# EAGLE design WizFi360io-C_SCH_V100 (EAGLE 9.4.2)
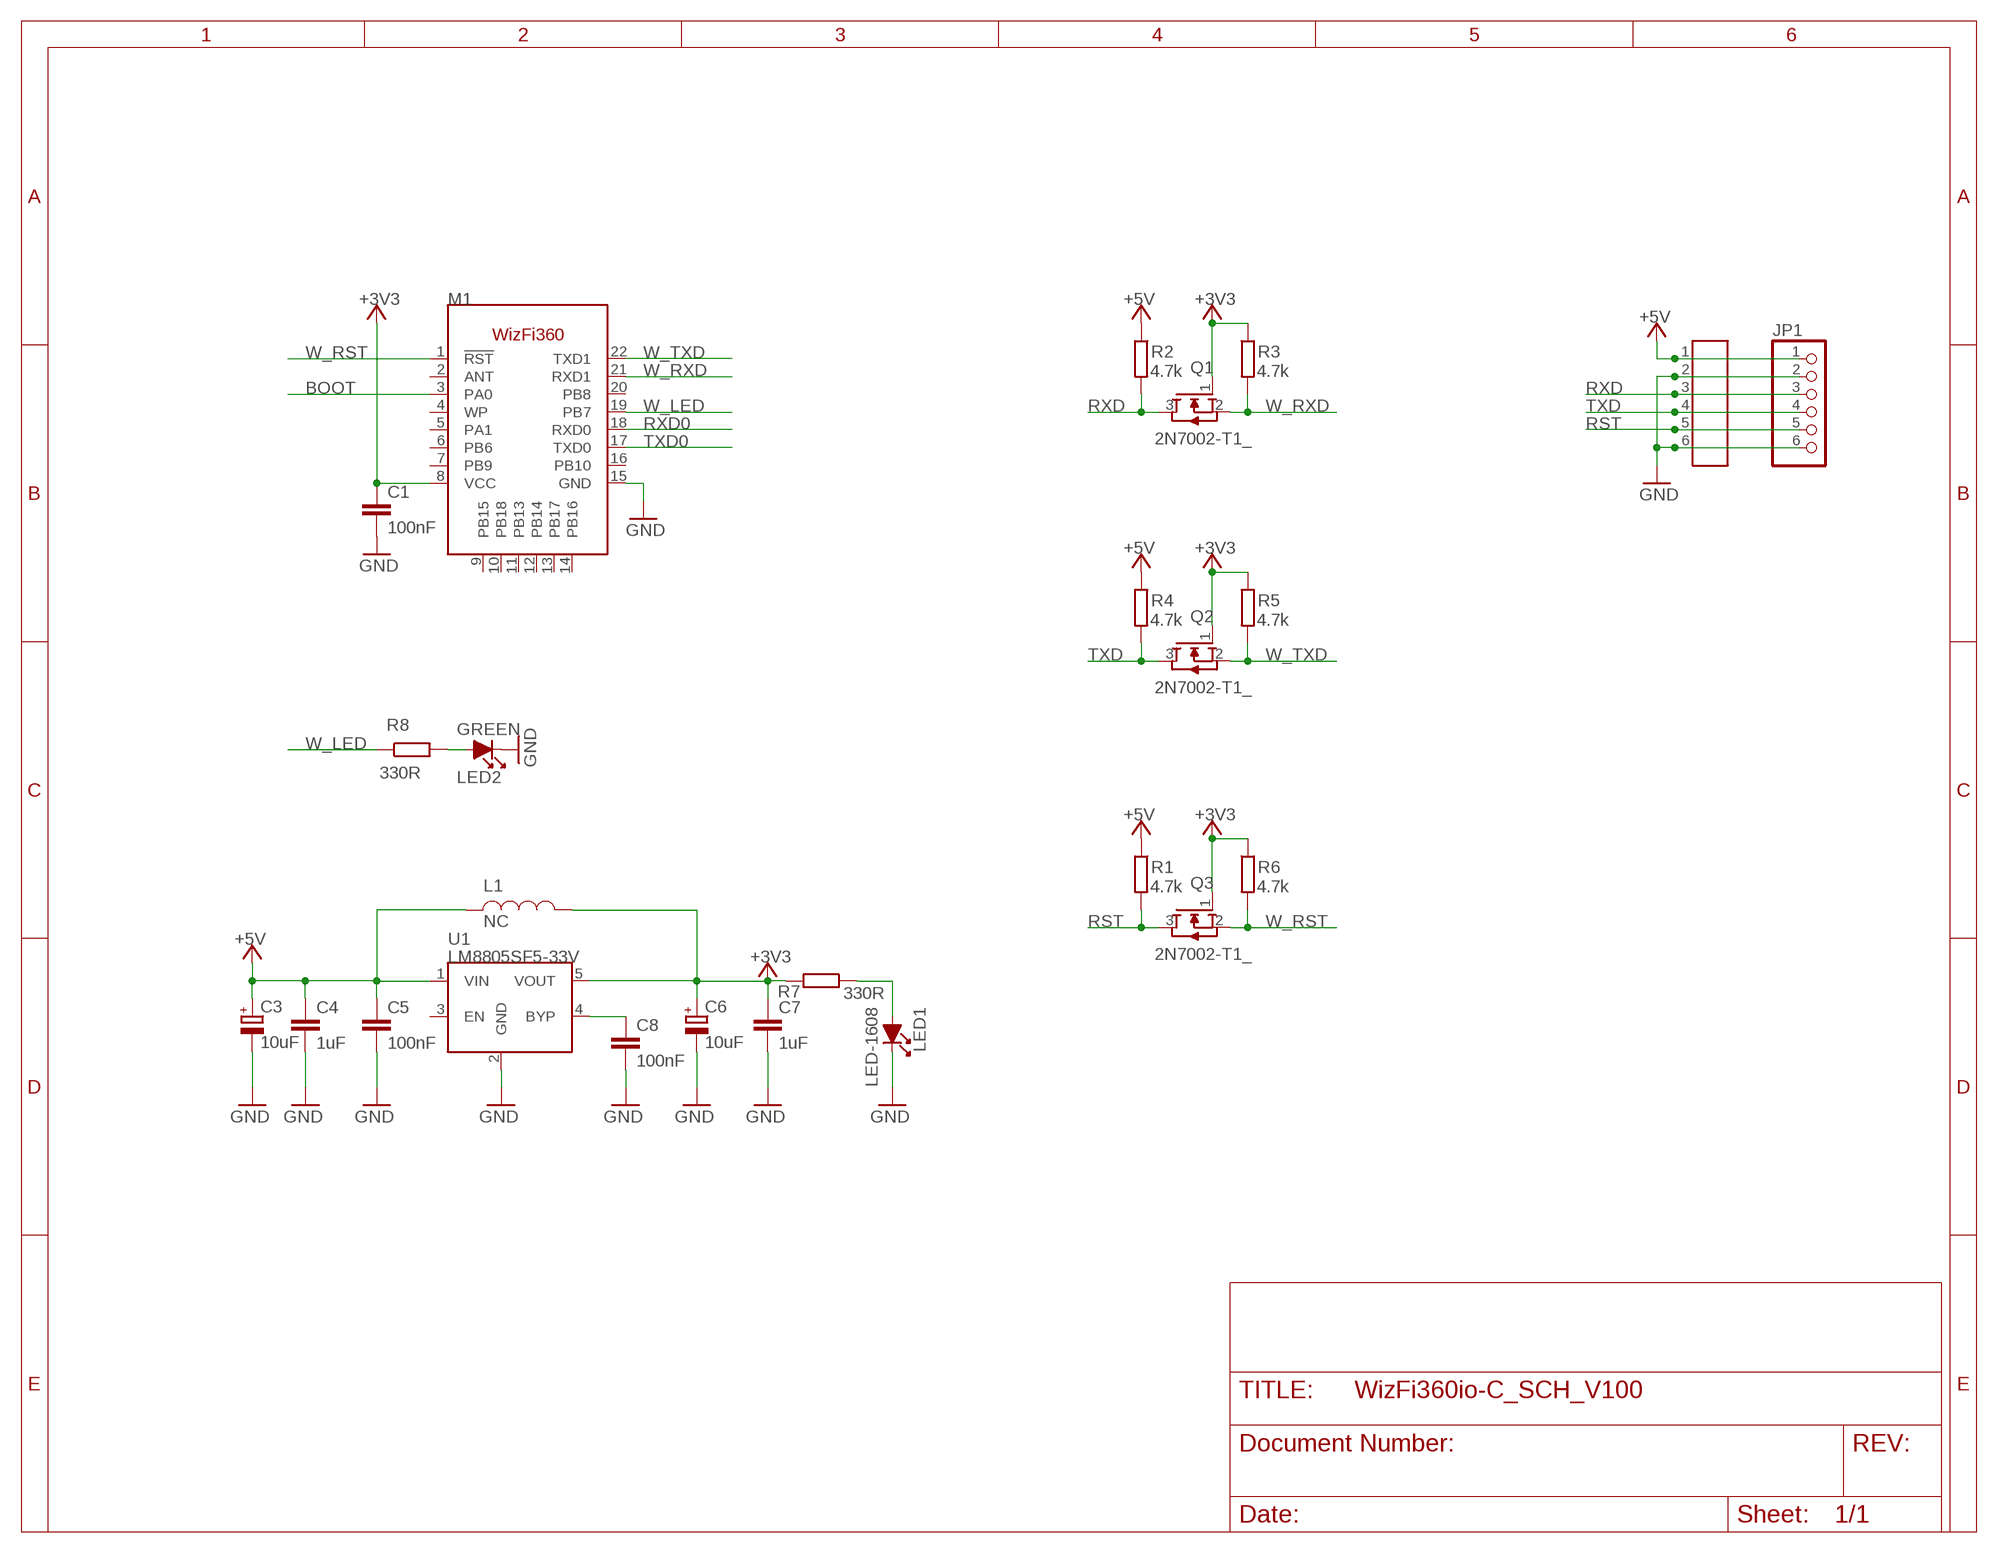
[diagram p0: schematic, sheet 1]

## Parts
C1  100nF  0142_10NF_0603  [C0603-ROUND@1]
C3  10uF  0474_TAJA475M016RNJ  [SMC_A]
C4  1uF  0142_10NF_0603  [C0603-ROUND@1]
C5  100nF  0142_10NF_0603  [C0603-ROUND@1]
C6  10uF  0474_TAJA475M016RNJ  [SMC_A]
C7  1uF  0142_10NF_0603  [C0603-ROUND@1]
C8  100nF  0142_10NF_0603  [C0603-ROUND@1]
JP1  PINHD-1X6NO_SILK  [1X06_NO_SILK]
JP4  SMW200-06  [SMW200-06]
L1  NC  L-1608  [L-1608]
LED1  LED-1608  [LED-1608]
LED2  GREEN  LED-1608  [LED-1608]
M1  WIZFI360  [WIZFI360]
Q1  2N7002-T1_  [SOT23]
Q2  2N7002-T1_  [SOT23]
Q3  2N7002-T1_  [SOT23]
R1  4.7k  0028_CR0603JW103L  [R0603-ROUND]
R2  4.7k  0028_CR0603JW103L  [R0603-ROUND]
R3  4.7k  0028_CR0603JW103L  [R0603-ROUND]
R4  4.7k  0028_CR0603JW103L  [R0603-ROUND]
R5  4.7k  0028_CR0603JW103L  [R0603-ROUND]
R6  4.7k  0028_CR0603JW103L  [R0603-ROUND]
R7  330R  0028_CR0603JW103L  [R0603-ROUND]
R8  330R  0028_CR0603JW103L  [R0603-ROUND]
U1  LM8805SF5-33V  [SOT23-5L]

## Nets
+3V3 [power]: C1.1 C6.+ C7.1 L1.P$2 M1.8(VCC) Q1.1(G) Q2.1(G) Q3.1(G) R3.1 R5.1 R6.1 R7.2 U1.5(VOUT)
+5V: C3.+ C4.1 C5.1 JP1.1 JP4.1 L1.1 R1.1 R2.1 R4.1 U1.1(VIN)
BOOT: M1.3(PA0)
GND: C1.2 C3.- C4.2 C5.2 C6.- C7.2 C8.2 JP1.2 JP1.6 JP4.2 JP4.6 LED1.K LED2.K M1.15(GND) U1.2(GND)
N$2: C8.1 U1.4(BYP)
N$7: LED1.A R7.1
N$17: LED2.A R8.2
RST: JP1.5 JP4.5 Q3.3(D) R1.2
RXD: JP1.3 JP4.3 Q1.3(D) R2.2
RXD0: M1.18(RXD0)
TXD: JP1.4 JP4.4 Q2.3(D) R4.2
TXD0: M1.17(TXD0)
W_LED: M1.19(PB7) R8.1
W_RST: M1.1(!RST!) Q3.2(S) R6.2
W_RXD: M1.21(RXD1) Q1.2(S) R3.2
W_TXD: M1.22(TXD1) Q2.2(S) R5.2
Unconnected: M1.2(ANT) M1.4(WP) M1.5(PA1) M1.6(PB6) M1.7(PB9) M1.9(PB15) M1.10(PB18) M1.11(PB13) M1.12(PB14) M1.13(PB17) M1.14(PB16) M1.16(PB10) M1.20(PB8) U1.3(EN)

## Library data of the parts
C1 C4 C5 C7 C8 = Condensatori:0142_10NF_0603: 10nF 0603; CASE: 0603; MONTHLY_USAGE: _____; PART_NUMBER: 10nF_0603; PRICE: _____; SUPPLIER: _____; TYPE: Condensatori; VALUE: 10nF
C3 C6 = Condensatori:0474_TAJA475M016RNJ: 4u7 tantalio Case A - testa gialla -Tantalio; CASE: CaseA_(1206); MONTHLY_USAGE: _____; PART_NUMBER: TAJA475M016RNJ; PRICE: _____; SUPPLIER: _____; TYPE: Condensatori; VALUE: 4u7
JP1 = PinHeader:PINHD-1X6: PIN HEADER
JP4 = Connector:SMW200-06
L1 = INDUCTOR:L-1608
LED1 LED2 = DIODE:LED-1608
M1 = WIZnet:WIZFI360
Q1-Q3 = TRANSISTOR:2N7002-T1
R1-R8 = Resistenze:0028_CR0603JW103L: 10K 0603; CASE: 0603; MONTHLY_USAGE: _____; PART_NUMBER: CR0603JW103L; PRICE: _____; SUPPLIER: _____; TYPE: Resistenze; VALUE: 10k
U1 = RECULATOR:LM8805SF5-33V

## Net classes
0 default: width 0.203 mm, drill 0.008 mm, clearance 0.127 mm
1 power: width 0.305 mm, drill 0.3 mm, clearance 0.203 mm

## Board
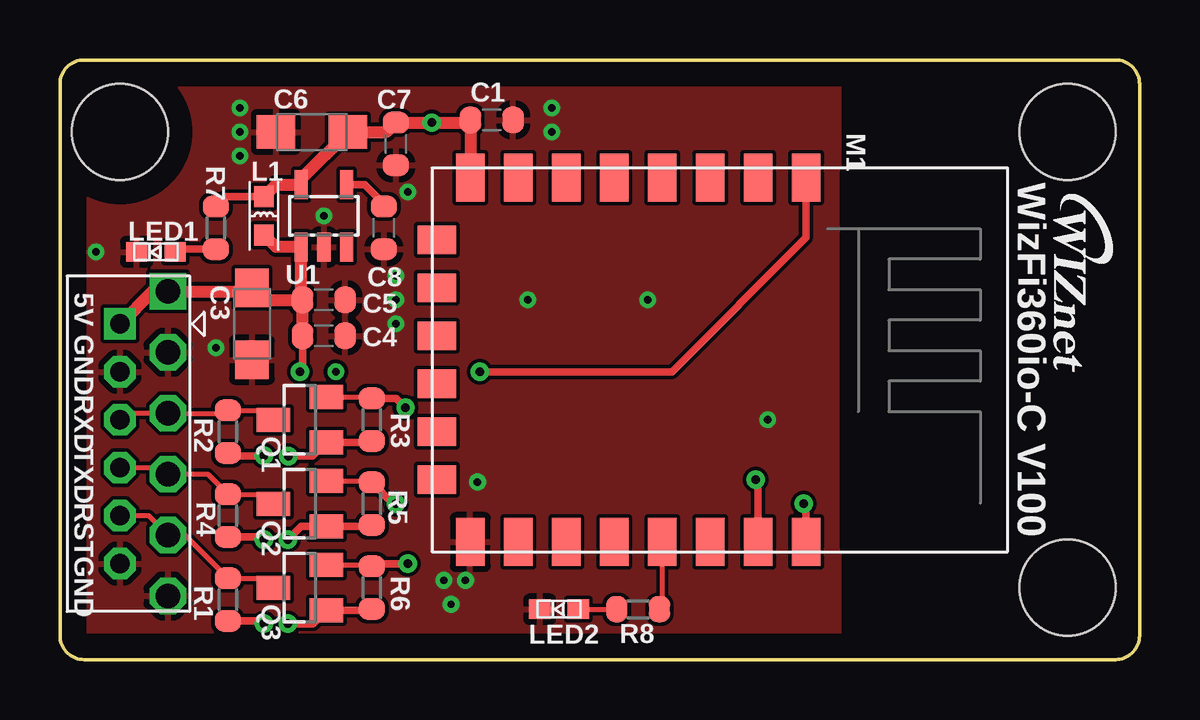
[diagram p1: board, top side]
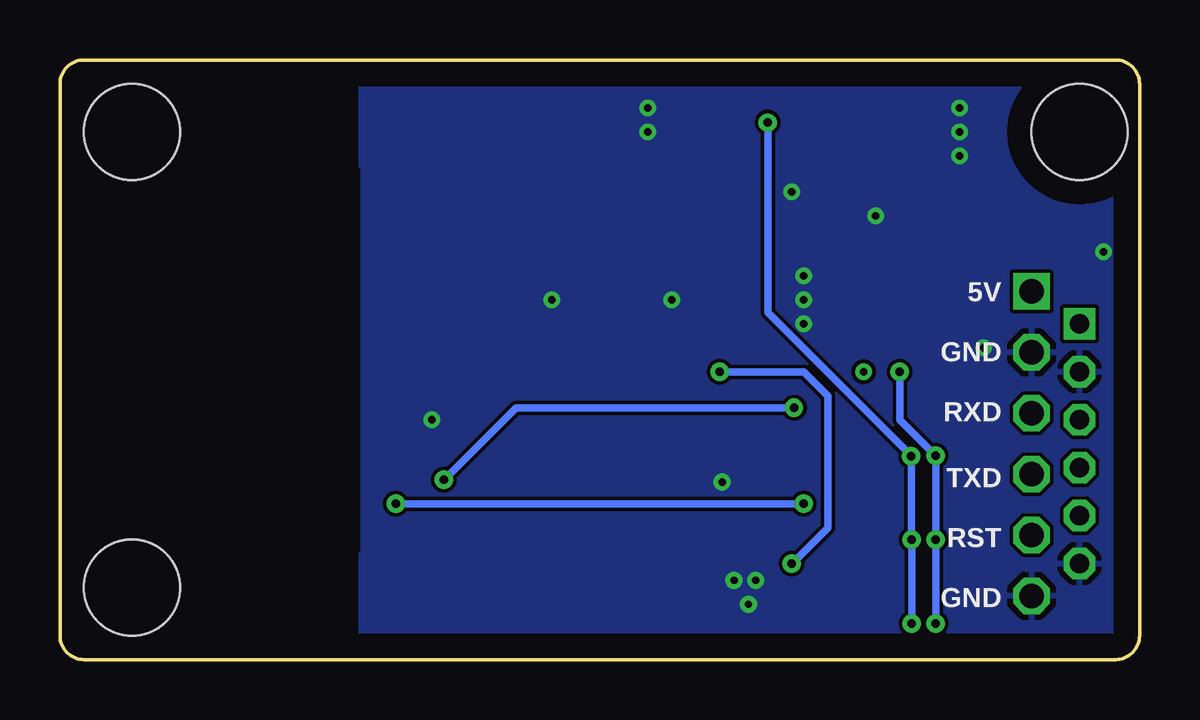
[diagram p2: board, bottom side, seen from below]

Size 45 x 25 mm. Coordinates in mm from the lower left corner, seen from the top.
Outline: 0,24 0,1 arc90 1,0 44,0 arc90 45,1 45,24 arc90 44,25 1,25 arc90 0,24
Copper layers (1*16): Top 0.035mm / dielectric 1.5mm / Bottom 0.035mm
Design rules "default *": minimum track width 6mil, minimum drill 0.35mm, track to track 6mil, track to pad 6mil, pad to pad 6mil, via to via 6mil, smd to smd 6mil, copper to edge 40mil, drill to drill 10mil, minimum pad ring 10mil, minimum via ring 8mil, stop-mask expansion 4mil, vias tented up to drill 15mil, thermal gap 10mil
Holes 4 mm at 2.5,22 42,22 42,3

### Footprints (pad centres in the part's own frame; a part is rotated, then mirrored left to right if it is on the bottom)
C0603-ROUND@1 = smd 0.898 x 1.1: 1 -0.889,0; 2 0.889,0
SMC_A = smd 1.6 x 1.4: + -1.5,0; - 1.5,0
1X06_NO_SILK = drill 1.016 square: 1 -6.35,0 | drill 1.016 octagon: 2 -3.81,0; 3 -1.27,0; 4 1.27,0; 5 3.81,0; 6 6.35,0
SMW200-06 = drill 0.8 square: 1 -5,0 | drill 0.8 octagon: 2 -3,0; 3 -1,0; 4 1,0; 5 3,0; 6 5,0
L-1608 = smd 0.89 x 0.82: 1 -0.8,0; P$2 0.8,0
LED-1608 = smd 0.89 x 0.82: A -0.8,0; K 0.8,0
WIZFI360 = smd 2 x 1.2: 1 -7.6,3.6; 2 -7.6,1.6; 3 -7.6,-0.4; 4 -7.6,-2.4; 5 -7.6,-4.4; 6 -7.6,-6.4; 7 -7.6,-8.4; 8 -7.6,-10.4; 15 7.6,-10.4; 16 7.6,-8.4; 17 7.6,-6.4; 18 7.6,-4.4; 19 7.6,-2.4; 20 7.6,-0.4; 21 7.6,1.6; 22 7.6,3.6 | smd 1.2 x 1.6: 9 -5,-11.8; 10 -3,-11.8; 11 -1,-11.8; 12 1,-11.8; 13 3,-11.8; 14 5,-11.8
SOT23 = smd 1 x 1.4: 1 -0.95,-1.1; 2 0.95,-1.1; 3 0,1.1
R0603-ROUND = smd 0.898 x 1.1: 1 -0.889,0; 2 0.889,0
SOT23-5L = smd 0.55 x 1.2: 1 -0.95,-1.3; 2 0,-1.3; 3 0.95,-1.3; 4 0.95,1.3; 5 -0.95,1.3

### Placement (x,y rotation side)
C1  18,22.5 0 top
C3  8,14 270 top
C4  11,13.5 0 top
C5  11,15 0 top
C6  10.5,22 180 top
C7  14,21.5 270 top
C8  13.5,18 270 top
JP1  4.5,9 270 top
JP4  2.5,9 270 top
L1  8.5,18.5 90 top
LED1  4,17 180 top
LED2  20.8,2.1 180 top
M1  27.5,12.5 270 top
Q1  10,10 90 top
Q2  10,6.5 90 top
Q3  10,3 90 top
R1  7,2.5 90 top
R2  7,9.5 90 top
R3  13,10 90 top
R4  7,6 90 top
R5  13,6.5 90 top
R6  13,3 90 top
R7  6.5,18 90 top
R8  24.1,2.1 180 top
U1  11,18.5 0 top
U$1  [WIZNET3-LOGO]  41.4,19.6 270 top

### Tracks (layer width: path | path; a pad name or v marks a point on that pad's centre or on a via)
+3V3  (via drill 0.35)
  Top 0.305: L1.P$2 6.91,19.3 R7.2 | R3.1 12.94,9.05 Q1.1 10.53,8.48 v9.52,8.48 | R5.1 12.94,5.55 Q2.1 10.05,5.55 v9.5,5 | R6.1 12.94,2.05 Q3.1 10.55,1.5 v9.5,1.5
  Top 0.508: L1.P$2 9,19.8 U1.5 10.05,20.05 C6.+ 13.61,22 C7.1 v15.5,22.39 17,22.39 C1.1 17.11,20.11 M1.8
  Bottom 0.305: v9.5,1.5 v9.5,5 9.52,5.02 v9.52,8.48 15.5,14.46 v15.5,22.39
+5V  (via drill 0.35)
  Top 0.305: C4.1 10.11,12.11 v10,12 | v8.5,8.5 7.11,8.5 R2.1 | R4.1 8.39,5.11 v8.5,5 | R1.1 8.39,1.61 v8.5,1.5
  Top 0.508: C4.1 C5.1 | C5.1 8.5,15 C3.+ 7.85,15.35 JP1.1 3.85,15.35 JP4.1 | C5.1 10.05,15.06 U1.1 9,17.2 L1.1
  Bottom 0.305: v10,12 10,10 v8.5,8.5 v8.5,5 v8.5,1.5
BOOT
  Top 0.203: M1.3 27.07,20.13
GND  (via drill 0.3)
  other vias: 16.9,3.3 16,3.3 16.3,2.3 17.4,7.4 29.5,10 24.5,15 19.5,15 14,15 14,14 14,16 14.5,19.5 11,18.5 20.5,22 20.5,23 7.5,21 7.5,22 7.5,23 1.5,17 6.5,13
  pour Top: 0,0 32.5,0 32.5,25 0,25
  pour Bottom: -1,-1 32.5,-1 32.5,26 -1,26
N$2
  Top 0.305: U1.4 12.7,19.8 13.5,19 C8.1
N$7
  Top 0.305: R7.1 4.91,17.11 LED1.A
N$17
  Top 0.203: LED2.A R8.2
N$23  (via drill 0.3)
  other vias: 11.5,12
RST
  Top 0.203: Q3.3 8.51,3.39 R1.2 5.2,5.19 JP1.5 3.69,6 JP4.5
RXD
  Top 0.203: 2.77,10.27 2.89,10.39 | Q1.3 8.51,10.39 R2.2 6.88,10.27 JP1.3 2.77,10.27 | 2.77,10.27 JP4.3
RXD0
  Top 0.203: 23.17,4.83 M1.18
TXD
  Top 0.203: Q2.3 8.51,6.89 R4.2 6.16,7.73 JP1.4 4.23,8 JP4.4
W_LED
  Top 0.203: M1.19 25.1,2.21 R8.1
W_RST  (via drill 0.35)
  Top 0.203: Q3.2 12.94,3.95 R6.2
  Top 0.305: R6.2 13.11,4 v14.5,4 | v17.5,12 25.5,12 31.1,17.6 M1.1
  Bottom 0.305: v14.5,4 13,5.5 13,11 14,12 v17.5,12
W_RXD  (via drill 0.35)
  Top 0.203: Q1.2 12.94,10.95 R3.2
  Top 0.305: R3.2 14.01,10.89 v14.4,10.5 | v29,7.5 29.1,7.4 M1.21
  Bottom 0.305: v14.4,10.5 26,10.5 v29,7.5
W_TXD  (via drill 0.35)
  Top 0.203: Q2.2 12.94,7.45 R5.2
  Top 0.305: R5.2 13.89,6.5 v14,6.5 | v31,6.5 31.1,6.4 M1.22
  Bottom 0.305: v14,6.5 v31,6.5

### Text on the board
tNames: 5V | GND | WizFi360io-C V100 | RXD | TXD | RST | GND
bNames: 5V | GND | RXD | TXD | RST | GND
